| Teraspeed Labs
| http://www.teraspeedlabs.com
[IBIS Ver]  4.0
[File Name] ev12as350a.ibs
[File Rev]  3.0
[Source]  Created by Teraspeed Labs
[Date]   02/10/2017
[Notes]   Quality Check of this IBIS model: Model Passes IBIS Check
   Model parses into ICX IS. Simulation done with Hyperlynx.
   1. MIN TYP MAX information is based on Temperature and
   Voltage characteristics only.
   2. Package data gained using Tektronix IConnect Software.
[Disclaimer]
| Use: Teraspeed Labs  ("Teraspeed") has
| licensed IBIS models to specific integrated circuit
| suppliers ("IC Vendors") for use and distribution as
| follows: Each IC Vendor may use IBIS Models, and distribute
| them to IC Vendor's customers to use solely for developing
| printed circuit board designs. Users of this model may
| modify the IBIS model to suit its specific applications but
| rights to derivative works and such modifications shall belong
| to Teraspeed. No other distribution of these materials is
| permitted.
| DISCLAIMER OF WARRANTY: UNLESS OTHERWISE AGREED TO IN WRITING
| TERASPEED DISCLAIMS AND USER WAIVES ALL WARRANTIES, EXPRESS
| OR IMPLIED, INCLUDING WARRANTIES OF MERCHANTABILITY AND
| FITNESS FOR A PARTICULAR PURPOSE. IN NO EVENT SHALL
| TERASPEED BE LIABLE FOR ANY DIRECT OR INDIRECT DAMAGES,
| WHETHER IN CONTRACT OR TORT, INCLUDING, WITHOUT LIMITATION,
| LOST PROFITS, BUSINESS INTERRUPTION, OR LOST INFORMATION
| ARISING OUT OF THE USE OF OR THE INABILITY TO USE THE MODEL,
| EVEN IF TERASPEED HAS BEEN ADVISED OF THE POSSIBILITY OF SUCH
| DAMAGES.
[Copyright]
| This file is the legal property of Teraspeed Labs Copyright(c) 2017.
| All other rights are reserved.
[Component]   EV12AS350A
[Manufacturer] e2v semiconductors
| Data Sheet: 1160DX-December 15
[Package]
| EBGA380 RoHS
| variable   typ   min   max
R_pkg  1.099E-02  6.371E-03  1.748E-02
L_pkg  2.017E-09  7.430E-10  5.787E-09
C_pkg  7.766E-13  4.120E-13  1.913E-12
[Pin] signal_name   model_name   R_pin   L_pin   C_pin
A1   GND   GND   1.748E-02   7.430E-10   4.120E-13
A2   VCCD   POWER   1.660E-02   7.430E-10   4.120E-13
A3   ABP   lvds_out   1.577E-02   5.787E-09   1.913E-12
A4   ADR   lvds_out   1.499E-02   5.500E-09   1.818E-12
A5   AIR   lvds_out   1.426E-02   5.234E-09   1.730E-12
A6   GND   GND   1.360E-02   7.430E-10   4.120E-13
A7   CMIREFAB   POWER   1.301E-02   7.430E-10   4.120E-13
A8   CMIREFCD   POWER   1.251E-02   7.430E-10   4.120E-13
A9   GND   GND   1.209E-02   7.430E-10   4.120E-13
A10   GND   GND   1.177E-02   7.430E-10   4.120E-13
A11   GND   GND   1.155E-02   7.430E-10   4.120E-13
A12   VIN   analog   1.144E-02   7.430E-10   4.120E-13
A13   VINN   analog   1.144E-02   7.430E-10   4.120E-13
A14   GND   GND   1.155E-02   7.430E-10   4.120E-13
A15   GND   GND   1.177E-02   7.430E-10   4.120E-13
A16   GND   GND   1.209E-02   7.430E-10   4.120E-13
A17   NC   NC   1.251E-02   7.430E-10   4.120E-13
A18   NC   NC   1.301E-02   7.430E-10   4.120E-13
A19   GND   GND   1.360E-02   7.430E-10   4.120E-13
A20   DIR   lvds_out   1.426E-02   5.234E-09   1.730E-12
A21   DDR   lvds_out   1.499E-02   5.500E-09   1.818E-12
A22   DBP   lvds_out   1.577E-02   5.787E-09   1.913E-12
A23   VCCD   POWER   1.660E-02   7.430E-10   4.120E-13
A24   GND   GND   1.748E-02   7.430E-10   4.120E-13
B1   GND   GND   1.660E-02   7.430E-10   4.120E-13
B2   VCCD   POWER   1.568E-02   7.430E-10   4.120E-13
B3   ABPN   lvds_out   1.481E-02   5.435E-09   1.797E-12
B4   ADRN   lvds_out   1.398E-02   5.131E-09   1.696E-12
B5   AIRN   lvds_out   1.321E-02   4.849E-09   1.603E-12
B6   GND   GND   1.251E-02   7.430E-10   4.120E-13
B7   GND   GND   1.188E-02   7.430E-10   4.120E-13
B8   GND   GND   1.133E-02   7.430E-10   4.120E-13
B9   GND   GND   1.088E-02   7.430E-10   4.120E-13
B10   GND   GND   1.053E-02   7.430E-10   4.120E-13
B11   GND   GND   1.030E-02   7.430E-10   4.120E-13
B12   GND   GND   1.018E-02   7.430E-10   4.120E-13
B13   GND   GND   1.018E-02   7.430E-10   4.120E-13
B14   GND   GND   1.030E-02   7.430E-10   4.120E-13
B15   GND   GND   1.053E-02   7.430E-10   4.120E-13
B16   GND   GND   1.088E-02   7.430E-10   4.120E-13
B17   GND   GND   1.133E-02   7.430E-10   4.120E-13
B18   GND   GND   1.188E-02   7.430E-10   4.120E-13
B19   GND   GND   1.251E-02   7.430E-10   4.120E-13
B20   DIRN   lvds_out   1.321E-02   4.849E-09   1.603E-12
B21   DDRN   lvds_out   1.398E-02   5.131E-09   1.696E-12
B22   DBPN   lvds_out   1.481E-02   5.435E-09   1.797E-12
B23   VCCD   POWER   1.568E-02   7.430E-10   4.120E-13
B24   GND   GND   1.660E-02   7.430E-10   4.120E-13
C1   A11   lvds_out   1.577E-02   5.787E-09   1.913E-12
C2   A11N   lvds_out   1.481E-02   5.435E-09   1.797E-12
C3   VCCD   POWER   1.389E-02   7.430E-10   4.120E-13
C4   GND   GND   1.301E-02   7.430E-10   4.120E-13
C5   VCCD   POWER   1.220E-02   7.430E-10   4.120E-13
C6   VCCD   POWER   1.144E-02   7.430E-10   4.120E-13
C7   GND   GND   1.077E-02   7.430E-10   4.120E-13
C8   GND   GND   1.018E-02   7.430E-10   4.120E-13
C9   GND   GND   9.683E-03   7.430E-10   4.120E-13
C10   GND   GND   9.301E-03   7.430E-10   4.120E-13
C11   GND   GND   9.040E-03   7.430E-10   4.120E-13
C12   GND   GND   8.907E-03   7.430E-10   4.120E-13
C13   GND   GND   8.907E-03   7.430E-10   4.120E-13
C14   GND   GND   9.040E-03   7.430E-10   4.120E-13
C15   GND   GND   9.301E-03   7.430E-10   4.120E-13
C16   GND   GND   9.683E-03   7.430E-10   4.120E-13
C17   GND   GND   1.018E-02   7.430E-10   4.120E-13
C18   GND   GND   1.077E-02   7.430E-10   4.120E-13
C19   VCCD   POWER   1.144E-02   7.430E-10   4.120E-13
C20   VCCD   POWER   1.220E-02   7.430E-10   4.120E-13
C21   GND   GND   1.301E-02   7.430E-10   4.120E-13
C22   VCCD   POWER   1.389E-02   7.430E-10   4.120E-13
C23   D11N   lvds_out   1.481E-02   5.435E-09   1.797E-12
C24   D11   lvds_out   1.577E-02   5.787E-09   1.913E-12
D1   A10   lvds_out   1.499E-02   5.500E-09   1.818E-12
D2   A10N   lvds_out   1.398E-02   5.131E-09   1.696E-12
D3   VCCD   POWER   1.301E-02   7.430E-10   4.120E-13
D4   GND   GND   1.209E-02   7.430E-10   4.120E-13
D5   VCCO1   POWER   1.122E-02   7.430E-10   4.120E-13
D6   VCCD   POWER   1.042E-02   7.430E-10   4.120E-13
D7   VCCD   POWER   9.683E-03   7.430E-10   4.120E-13
D8   GND   GND   9.040E-03   7.430E-10   4.120E-13
D9   GND   GND   8.499E-03   7.430E-10   4.120E-13
D10   GND   GND   8.077E-03   7.430E-10   4.120E-13
D11   GND   GND   7.787E-03   7.430E-10   4.120E-13
D12   GND   GND   7.639E-03   7.430E-10   4.120E-13
D13   GND   GND   7.639E-03   7.430E-10   4.120E-13
D14   GND   GND   7.787E-03   7.430E-10   4.120E-13
D15   GND   GND   8.077E-03   7.430E-10   4.120E-13
D16   GND   GND   8.499E-03   7.430E-10   4.120E-13
D17   GND   GND   9.040E-03   7.430E-10   4.120E-13
D18   VCCD   POWER   9.683E-03   7.430E-10   4.120E-13
D19   VCCD   POWER   1.042E-02   7.430E-10   4.120E-13
D20   VCCO1   POWER   1.122E-02   7.430E-10   4.120E-13
D21   GND   GND   1.209E-02   7.430E-10   4.120E-13
D22   VCCD   POWER   1.301E-02   7.430E-10   4.120E-13
D23   D10N   lvds_out   1.398E-02   5.131E-09   1.696E-12
D24   D10   lvds_out   1.499E-02   5.500E-09   1.818E-12
E1   A9   lvds_out   1.426E-02   5.234E-09   1.730E-12
E2   A9N   lvds_out   1.321E-02   4.849E-09   1.603E-12
E3   VCCO1   POWER   1.220E-02   7.430E-10   4.120E-13
E4   GNDO   GND   1.122E-02   7.430E-10   4.120E-13
E5   GNDO   GND   1.030E-02   7.430E-10   4.120E-13
E6   VCCO1   POWER   9.429E-03   7.430E-10   4.120E-13
E7   VCCD   POWER   8.637E-03   7.430E-10   4.120E-13
E8   GND   GND   7.933E-03   7.430E-10   4.120E-13
E9   GND   GND   7.336E-03   7.430E-10   4.120E-13
E10   GND   GND   6.865E-03   7.430E-10   4.120E-13
E11   GND   GND   6.539E-03   7.430E-10   4.120E-13
E12   GND   GND   6.371E-03   7.430E-10   4.120E-13
E13   GND   GND   6.371E-03   7.430E-10   4.120E-13
E14   GND   GND   6.539E-03   7.430E-10   4.120E-13
E15   GND   GND   6.865E-03   7.430E-10   4.120E-13
E16   GND   GND   7.336E-03   7.430E-10   4.120E-13
E17   GND   GND   7.933E-03   7.430E-10   4.120E-13
E18   VCCD   POWER   8.637E-03   7.430E-10   4.120E-13
E19   VCCO1   POWER   9.429E-03   7.430E-10   4.120E-13
E20   GNDO   GND   1.030E-02   7.430E-10   4.120E-13
E21   GNDO   GND   1.122E-02   7.430E-10   4.120E-13
E22   VCCO1   POWER   1.220E-02   7.430E-10   4.120E-13
E23   D9N   lvds_out   1.321E-02   4.849E-09   1.603E-12
E24   D9   lvds_out   1.426E-02   5.234E-09   1.730E-12
F1   A8   lvds_out   1.360E-02   4.992E-09   1.650E-12
F2   A8N   lvds_out   1.251E-02   4.591E-09   1.518E-12
F3   VCCO1   POWER   1.144E-02   7.430E-10   4.120E-13
F4   GNDO   GND   1.042E-02   7.430E-10   4.120E-13
F5   GNDO   GND   9.429E-03   7.430E-10   4.120E-13
F20   GNDO   GND   9.429E-03   7.430E-10   4.120E-13
F21   GNDO   GND   1.042E-02   7.430E-10   4.120E-13
F22   VCCO1   POWER   1.144E-02   7.430E-10   4.120E-13
F23   D8N   lvds_out   1.251E-02   4.591E-09   1.518E-12
F24   D8   lvds_out   1.360E-02   4.992E-09   1.650E-12
G1   A6   lvds_out   1.301E-02   4.776E-09   1.579E-12
G2   A6N   lvds_out   1.188E-02   4.359E-09   1.441E-12
G3   A7   lvds_out   1.077E-02   3.951E-09   1.306E-12
G4   A7N   lvds_out   9.683E-03   3.554E-09   1.175E-12
G5   GNDO   GND   8.637E-03   7.430E-10   4.120E-13
G20   GNDO   GND   8.637E-03   7.430E-10   4.120E-13
G21   D7N   lvds_out   9.683E-03   3.554E-09   1.175E-12
G22   D7   lvds_out   1.077E-02   3.951E-09   1.306E-12
G23   D6N   lvds_out   1.188E-02   4.359E-09   1.441E-12
G24   D6   lvds_out   1.301E-02   4.776E-09   1.579E-12
H1   A4   lvds_out   1.251E-02   4.591E-09   1.518E-12
H2   A4N   lvds_out   1.133E-02   4.159E-09   1.375E-12
H3   A5   lvds_out   1.018E-02   3.734E-09   1.235E-12
H4   A5N   lvds_out   9.040E-03   3.318E-09   1.097E-12
H5   VCCO1   POWER   7.933E-03   7.430E-10   4.120E-13
H20   VCCO1   POWER   7.933E-03   7.430E-10   4.120E-13
H21   D5N   lvds_out   9.040E-03   3.318E-09   1.097E-12
H22   D5   lvds_out   1.018E-02   3.734E-09   1.235E-12
H23   D4N   lvds_out   1.133E-02   4.159E-09   1.375E-12
H24   D4   lvds_out   1.251E-02   4.591E-09   1.518E-12
J1   A2   lvds_out   1.209E-02   4.438E-09   1.467E-12
J2   A2N   lvds_out   1.088E-02   3.993E-09   1.320E-12
J3   A3   lvds_out   9.683E-03   3.554E-09   1.175E-12
J4   A3N   lvds_out   8.499E-03   3.119E-09   1.031E-12
J5   GND   GND   7.336E-03   7.430E-10   4.120E-13
J20   GND   GND   7.336E-03   7.430E-10   4.120E-13
J21   D3N   lvds_out   8.499E-03   3.119E-09   1.031E-12
J22   D3   lvds_out   9.683E-03   3.554E-09   1.175E-12
J23   D2N   lvds_out   1.088E-02   3.993E-09   1.320E-12
J24   D2   lvds_out   1.209E-02   4.438E-09   1.467E-12
K1   A0   lvds_out   1.177E-02   4.320E-09   1.428E-12
K2   A0N   lvds_out   1.053E-02   3.866E-09   1.278E-12
K3   A1   lvds_out   9.301E-03   3.413E-09   1.128E-12
K4   A1N   lvds_out   8.077E-03   2.964E-09   9.799E-13
K5   VCCD   POWER   6.865E-03   7.430E-10   4.120E-13
K20   VCCD   POWER   6.865E-03   7.430E-10   4.120E-13
K21   D1N   lvds_out   8.077E-03   2.964E-09   9.799E-13
K22   D1   lvds_out   9.301E-03   3.413E-09   1.128E-12
K23   D0N   lvds_out   1.053E-02   3.866E-09   1.278E-12
K24   D0   lvds_out   1.177E-02   4.320E-09   1.428E-12
L1   GND   GND   1.155E-02   7.430E-10   4.120E-13
L2   GND   GND   1.030E-02   7.430E-10   4.120E-13
L3   NC   NC   9.040E-03   7.430E-10   4.120E-13
L4   GND   GND   7.787E-03   7.430E-10   4.120E-13
L5   VCCD   POWER   6.539E-03   7.430E-10   4.120E-13
L20   VCCD   POWER   6.539E-03   7.430E-10   4.120E-13
L21   GND   GND   7.787E-03   7.430E-10   4.120E-13
L22   NC   NC   9.040E-03   7.430E-10   4.120E-13
L23   GND   GND   1.030E-02   7.430E-10   4.120E-13
L24   GND   GND   1.155E-02   7.430E-10   4.120E-13
M1   VCCA   POWER   1.144E-02   7.430E-10   4.120E-13
M2   GND   GND   1.018E-02   7.430E-10   4.120E-13
M3   VCCA   POWER   8.907E-03   7.430E-10   4.120E-13
M4   GND   GND   7.639E-03   7.430E-10   4.120E-13
M5   VCCD   POWER   6.371E-03   7.430E-10   4.120E-13
M20   VCCD   POWER   6.371E-03   7.430E-10   4.120E-13
M21   GND   GND   7.639E-03   7.430E-10   4.120E-13
M22   VCCA   POWER   8.907E-03   7.430E-10   4.120E-13
M23   GND   GND   1.018E-02   7.430E-10   4.120E-13
M24   VCCA   POWER   1.144E-02   7.430E-10   4.120E-13
N1   VCCA   POWER   1.144E-02   7.430E-10   4.120E-13
N2   GND   GND   1.018E-02   7.430E-10   4.120E-13
N3   VCCA   POWER   8.907E-03   7.430E-10   4.120E-13
N4   GND   GND   7.639E-03   7.430E-10   4.120E-13
N5   VCCD   POWER   6.371E-03   7.430E-10   4.120E-13
N20   VCCD   POWER   6.371E-03   7.430E-10   4.120E-13
N21   GND   GND   7.639E-03   7.430E-10   4.120E-13
N22   VCCA   POWER   8.907E-03   7.430E-10   4.120E-13
N23   GND   GND   1.018E-02   7.430E-10   4.120E-13
N24   VCCA   POWER   1.144E-02   7.430E-10   4.120E-13
P1   GND   GND   1.155E-02   7.430E-10   4.120E-13
P2   GND   GND   1.030E-02   7.430E-10   4.120E-13
P3   NC   NC   9.040E-03   7.430E-10   4.120E-13
P4   GND   GND   7.787E-03   7.430E-10   4.120E-13
P5   VCCD   POWER   6.539E-03   7.430E-10   4.120E-13
P20   VCCD   POWER   6.539E-03   7.430E-10   4.120E-13
P21   GND   GND   7.787E-03   7.430E-10   4.120E-13
P22   NC   NC   9.040E-03   7.430E-10   4.120E-13
P23   GND   GND   1.030E-02   7.430E-10   4.120E-13
P24   GND   GND   1.155E-02   7.430E-10   4.120E-13
R1   B0   lvds_out   1.177E-02   4.320E-09   1.428E-12
R2   B0N   lvds_out   1.053E-02   3.866E-09   1.278E-12
R3   B1   lvds_out   9.301E-03   3.413E-09   1.128E-12
R4   B1N   lvds_out   8.077E-03   2.964E-09   9.799E-13
R5   VCCD   POWER   6.865E-03   7.430E-10   4.120E-13
R20   VCCD   POWER   6.865E-03   7.430E-10   4.120E-13
R21   C1N   lvds_out   8.077E-03   2.964E-09   9.799E-13
R22   C1   lvds_out   9.301E-03   3.413E-09   1.128E-12
R23   C0N   lvds_out   1.053E-02   3.866E-09   1.278E-12
R24   C0   lvds_out   1.177E-02   4.320E-09   1.428E-12
T1   B2   lvds_out   1.209E-02   4.438E-09   1.467E-12
T2   B2N   lvds_out   1.088E-02   3.993E-09   1.320E-12
T3   B3   lvds_out   9.683E-03   3.554E-09   1.175E-12
T4   B3N   lvds_out   8.499E-03   3.119E-09   1.031E-12
T5   GND   GND   7.336E-03   7.430E-10   4.120E-13
T20   GND   GND   7.336E-03   7.430E-10   4.120E-13
T21   C3N   lvds_out   8.499E-03   3.119E-09   1.031E-12
T22   C3   lvds_out   9.683E-03   3.554E-09   1.175E-12
T23   C2N   lvds_out   1.088E-02   3.993E-09   1.320E-12
T24   C2   lvds_out   1.209E-02   4.438E-09   1.467E-12
U1   B4   lvds_out   1.251E-02   4.591E-09   1.518E-12
U2   B4N   lvds_out   1.133E-02   4.159E-09   1.375E-12
U3   B5   lvds_out   1.018E-02   3.734E-09   1.235E-12
U4   B5N   lvds_out   9.040E-03   3.318E-09   1.097E-12
U5   VCCO1   POWER   7.933E-03   7.430E-10   4.120E-13
U20   VCCO1   POWER   7.933E-03   7.430E-10   4.120E-13
U21   C5N   lvds_out   9.040E-03   3.318E-09   1.097E-12
U22   C5   lvds_out   1.018E-02   3.734E-09   1.235E-12
U23   C4N   lvds_out   1.133E-02   4.159E-09   1.375E-12
U24   C4   lvds_out   1.251E-02   4.591E-09   1.518E-12
V1   B6   lvds_out   1.301E-02   4.776E-09   1.579E-12
V2   B6N   lvds_out   1.188E-02   4.359E-09   1.441E-12
V3   B7   lvds_out   1.077E-02   3.951E-09   1.306E-12
V4   B7N   lvds_out   9.683E-03   3.554E-09   1.175E-12
V5   GNDO   GND   8.637E-03   7.430E-10   4.120E-13
V20   GNDO   GND   8.637E-03   7.430E-10   4.120E-13
V21   C7N   lvds_out   9.683E-03   3.554E-09   1.175E-12
V22   C7   lvds_out   1.077E-02   3.951E-09   1.306E-12
V23   C6N   lvds_out   1.188E-02   4.359E-09   1.441E-12
V24   C6   lvds_out   1.301E-02   4.776E-09   1.579E-12
W1   B8   lvds_out   1.360E-02   4.992E-09   1.650E-12
W2   B8N   lvds_out   1.251E-02   4.591E-09   1.518E-12
W3   VCCO1   POWER   1.144E-02   7.430E-10   4.120E-13
W4   GNDO   GND   1.042E-02   7.430E-10   4.120E-13
W5   GNDO   GND   9.429E-03   7.430E-10   4.120E-13
W20   GNDO   GND   9.429E-03   7.430E-10   4.120E-13
W21   GNDO   GND   1.042E-02   7.430E-10   4.120E-13
W22   VCCO1   POWER   1.144E-02   7.430E-10   4.120E-13
W23   C8N   lvds_out   1.251E-02   4.591E-09   1.518E-12
W24   C8   lvds_out   1.360E-02   4.992E-09   1.650E-12
Y1   B9   lvds_out   1.426E-02   5.234E-09   1.730E-12
Y2   B9N   lvds_out   1.321E-02   4.849E-09   1.603E-12
Y3   VCCO1   POWER   1.220E-02   7.430E-10   4.120E-13
Y4   GNDO   GND   1.122E-02   7.430E-10   4.120E-13
Y5   GNDO   GND   1.030E-02   7.430E-10   4.120E-13
Y6   VCCO1   POWER   9.429E-03   7.430E-10   4.120E-13
Y7   VCCD   POWER   8.637E-03   7.430E-10   4.120E-13
Y8   GND   GND   7.933E-03   7.430E-10   4.120E-13
Y9   GND   GND   7.336E-03   7.430E-10   4.120E-13
Y10   VCCD   POWER   6.865E-03   7.430E-10   4.120E-13
Y11   VCCD   POWER   6.539E-03   7.430E-10   4.120E-13
Y12   GND   GND   6.371E-03   7.430E-10   4.120E-13
Y13   GND   GND   6.371E-03   7.430E-10   4.120E-13
Y14   VCCD   POWER   6.539E-03   7.430E-10   4.120E-13
Y15   VCCD   POWER   6.865E-03   7.430E-10   4.120E-13
Y16   GND   GND   7.336E-03   7.430E-10   4.120E-13
Y17   GND   GND   7.933E-03   7.430E-10   4.120E-13
Y18   VCCD   POWER   8.637E-03   7.430E-10   4.120E-13
Y19   VCCO1   POWER   9.429E-03   7.430E-10   4.120E-13
Y20   GNDO   GND   1.030E-02   7.430E-10   4.120E-13
Y21   GNDO   GND   1.122E-02   7.430E-10   4.120E-13
Y22   VCCO1   POWER   1.220E-02   7.430E-10   4.120E-13
Y23   C9N   lvds_out   1.321E-02   4.849E-09   1.603E-12
Y24   C9   lvds_out   1.426E-02   5.234E-09   1.730E-12
AA1   B10   lvds_out   1.499E-02   5.500E-09   1.818E-12
AA2   B10N   lvds_out   1.398E-02   5.131E-09   1.696E-12
AA3   VCCD   POWER   1.301E-02   7.430E-10   4.120E-13
AA4   GND   GND   1.209E-02   7.430E-10   4.120E-13
AA5   VCCO1   POWER   1.122E-02   7.430E-10   4.120E-13
AA6   VCCD   POWER   1.042E-02   7.430E-10   4.120E-13
AA7   VCCD   POWER   9.683E-03   7.430E-10   4.120E-13
AA8   GND   GND   9.040E-03   7.430E-10   4.120E-13
AA9   GND   GND   8.499E-03   7.430E-10   4.120E-13
AA10   VCCD   POWER   8.077E-03   7.430E-10   4.120E-13
AA11   VCCD   POWER   7.787E-03   7.430E-10   4.120E-13
AA12   GND   GND   7.639E-03   7.430E-10   4.120E-13
AA13   GND   GND   7.639E-03   7.430E-10   4.120E-13
AA14   VCCD   POWER   7.787E-03   7.430E-10   4.120E-13
AA15   VCCD   POWER   8.077E-03   7.430E-10   4.120E-13
AA16   GND   GND   8.499E-03   7.430E-10   4.120E-13
AA17   GND   GND   9.040E-03   7.430E-10   4.120E-13
AA18   VCCD   POWER   9.683E-03   7.430E-10   4.120E-13
AA19   VCCD   POWER   1.042E-02   7.430E-10   4.120E-13
AA20   VCCO1   POWER   1.122E-02   7.430E-10   4.120E-13
AA21   GND   GND   1.209E-02   7.430E-10   4.120E-13
AA22   VCCD   POWER   1.301E-02   7.430E-10   4.120E-13
AA23   C10N   lvds_out   1.398E-02   5.131E-09   1.696E-12
AA24   C10   lvds_out   1.499E-02   5.500E-09   1.818E-12
AB1   B11   lvds_out   1.577E-02   5.787E-09   1.913E-12
AB2   B11N   lvds_out   1.481E-02   5.435E-09   1.797E-12
AB3   VCCD   POWER   1.389E-02   7.430E-10   4.120E-13
AB4   GND   GND   1.301E-02   7.430E-10   4.120E-13
AB5   VCCD   POWER   1.220E-02   7.430E-10   4.120E-13
AB6   GND   GND   1.144E-02   7.430E-10   4.120E-13
AB7   VCCD   POWER   1.077E-02   7.430E-10   4.120E-13
AB8   GND   GND   1.018E-02   7.430E-10   4.120E-13
AB9   GND   GND   9.683E-03   7.430E-10   4.120E-13
AB10   VCCD   POWER   9.301E-03   7.430E-10   4.120E-13
AB11   VCCD   POWER   9.040E-03   7.430E-10   4.120E-13
AB12   GND   GND   8.907E-03   7.430E-10   4.120E-13
AB13   GND   GND   8.907E-03   7.430E-10   4.120E-13
AB14   VCCD   POWER   9.040E-03   7.430E-10   4.120E-13
AB15   VCCD   POWER   9.301E-03   7.430E-10   4.120E-13
AB16   GND   GND   9.683E-03   7.430E-10   4.120E-13
AB17   GND   GND   1.018E-02   7.430E-10   4.120E-13
AB18   VCCD   POWER   1.077E-02   7.430E-10   4.120E-13
AB19   GND   GND   1.144E-02   7.430E-10   4.120E-13
AB20   VCCD   POWER   1.220E-02   7.430E-10   4.120E-13
AB21   GND   GND   1.301E-02   7.430E-10   4.120E-13
AB22   VCCD   POWER   1.389E-02   7.430E-10   4.120E-13
AB23   C11N   lvds_out   1.481E-02   5.435E-09   1.797E-12
AB24   C11   lvds_out   1.577E-02   5.787E-09   1.913E-12
AC1   GND   GND   1.660E-02   7.430E-10   4.120E-13
AC2   VCCD   POWER   1.568E-02   7.430E-10   4.120E-13
AC3   BBPN   lvds_out   1.481E-02   5.435E-09   1.797E-12
AC4   BDRN   lvds_out   1.398E-02   5.131E-09   1.696E-12
AC5   BIRN   lvds_out   1.321E-02   4.849E-09   1.603E-12
AC6   GND   GND   1.251E-02   7.430E-10   4.120E-13
AC7   diodeC   GND   1.188E-02   7.430E-10   4.120E-13
AC8   NC   NC   1.133E-02   7.430E-10   4.120E-13
AC9   GND   GND   1.088E-02   7.430E-10   4.120E-13
AC10   SYNCN   sync_in   1.053E-02   3.866E-09   1.278E-12
AC11   GND   GND   1.030E-02   7.430E-10   4.120E-13
AC12   GND   GND   1.018E-02   7.430E-10   4.120E-13
AC13   GND   GND   1.018E-02   7.430E-10   4.120E-13
AC14   GND   GND   1.030E-02   7.430E-10   4.120E-13
AC15   *RST   in_pu   1.053E-02   3.866E-09   1.278E-12
AC16   *CS   in_pu   1.088E-02   3.993E-09   1.320E-12
AC17   MISO   spi_out   1.133E-02   4.159E-09   1.375E-12
AC18   VCCO2   POWER   1.188E-02   7.430E-10   4.120E-13
AC19   GND   GND   1.251E-02   7.430E-10   4.120E-13
AC20   CIRN   lvds_out   1.321E-02   4.849E-09   1.603E-12
AC21   CDRN   lvds_out   1.398E-02   5.131E-09   1.696E-12
AC22   CBPN   lvds_out   1.481E-02   5.435E-09   1.797E-12
AC23   VCCD   POWER   1.568E-02   7.430E-10   4.120E-13
AC24   GND   GND   1.660E-02   7.430E-10   4.120E-13
AD1   GND   GND   1.748E-02   7.430E-10   4.120E-13
AD2   VCCD   POWER   1.660E-02   7.430E-10   4.120E-13
AD3   BBP   lvds_out   1.577E-02   5.787E-09   1.913E-12
AD4   BDR   lvds_out   1.499E-02   5.500E-09   1.818E-12
AD5   BIR   lvds_out   1.426E-02   5.234E-09   1.730E-12
AD6   GND   GND   1.360E-02   7.430E-10   4.120E-13
AD7   diodeA   NC   1.301E-02   7.430E-10   4.120E-13
AD8   GND   GND   1.251E-02   7.430E-10   4.120E-13
AD9   GND   GND   1.209E-02   7.430E-10   4.120E-13
AD10   SYNCP   sync_in   1.177E-02   4.320E-09   1.428E-12
AD11   GND   GND   1.155E-02   7.430E-10   4.120E-13
AD12   CLK   clk_in   1.144E-02   4.200E-09   1.388E-12
AD13   CLKN   clk_in   1.144E-02   4.200E-09   1.388E-12
AD14   GND   GND   1.155E-02   7.430E-10   4.120E-13
AD15   NC   NC   1.177E-02   7.430E-10   4.120E-13
AD16   SCLK   spi_in   1.209E-02   4.438E-09   1.467E-12
AD17   MOSI   spi_in   1.251E-02   4.591E-09   1.518E-12
AD18   VCCO2   POWER   1.301E-02   7.430E-10   4.120E-13
AD19   GND   GND   1.360E-02   7.430E-10   4.120E-13
AD20   CIR   lvds_out   1.426E-02   5.234E-09   1.730E-12
AD21   CDR   lvds_out   1.499E-02   5.500E-09   1.818E-12
AD22   CBP   lvds_out   1.577E-02   5.787E-09   1.913E-12
AD23   VCCD   POWER   1.660E-02   7.430E-10   4.120E-13
AD24   GND   GND   1.748E-02   7.430E-10   4.120E-13
[Diff Pin] inv_pin vdiff tdelay_typ tdelay_min tdelay_max
AD12   AD13   158mV   NA   NA   NA
AD10   AC10   100mV   NA   NA   NA
K1   K2   NA   NA   NA   NA
K3   K4   NA   NA   NA   NA
J1   J2   NA   NA   NA   NA
J3   J4   NA   NA   NA   NA
H1   H2   NA   NA   NA   NA
H3   H4   NA   NA   NA   NA
G1   G2   NA   NA   NA   NA
G3   G4   NA   NA   NA   NA
F1   F2   NA   NA   NA   NA
E1   E2   NA   NA   NA   NA
D1   D2   NA   NA   NA   NA
C1   C2   NA   NA   NA   NA
A3   B3   NA   NA   NA   NA
A5   B5   NA   NA   NA   NA
A4   B4   NA   NA   NA   NA
R1   R2   NA   NA   NA   NA
R3   R4   NA   NA   NA   NA
T1   T2   NA   NA   NA   NA
T3   T4   NA   NA   NA   NA
U1   U2   NA   NA   NA   NA
U3   U4   NA   NA   NA   NA
V1   V2   NA   NA   NA   NA
V3   V4   NA   NA   NA   NA
W1   W2   NA   NA   NA   NA
Y1   Y2   NA   NA   NA   NA
AA1   AA2   NA   NA   NA   NA
AB1   AB2   NA   NA   NA   NA
AD3   AC3   NA   NA   NA   NA
AD5   AC5   NA   NA   NA   NA
AD4   AC4   NA   NA   NA   NA
R24   R23   NA   NA   NA   NA
R22   R21   NA   NA   NA   NA
T24   T23   NA   NA   NA   NA
T22   T21   NA   NA   NA   NA
U24   U23   NA   NA   NA   NA
U22   U21   NA   NA   NA   NA
V24   V23   NA   NA   NA   NA
V22   V21   NA   NA   NA   NA
W24   W23   NA   NA   NA   NA
Y24   Y23   NA   NA   NA   NA
AA24   AA23   NA   NA   NA   NA
AB24   AB23   NA   NA   NA   NA
AD22   AC22   NA   NA   NA   NA
AD20   AC20   NA   NA   NA   NA
AD21   AC21   NA   NA   NA   NA
K24   K23   NA   NA   NA   NA
K22   K21   NA   NA   NA   NA
J24   J23   NA   NA   NA   NA
J22   J21   NA   NA   NA   NA
H24   H23   NA   NA   NA   NA
H22   H21   NA   NA   NA   NA
G24   G23   NA   NA   NA   NA
G22   G21   NA   NA   NA   NA
F24   F23   NA   NA   NA   NA
E24   E23   NA   NA   NA   NA
D24   D23   NA   NA   NA   NA
C24   C23   NA   NA   NA   NA
A22   B22   NA   NA   NA   NA
A20   B20   NA   NA   NA   NA
A21   B21   NA   NA   NA   NA
[Series Pin Mapping] pin_2 model_name function_table_group
AD12   AD13   100ohm
AD10   AC10   100ohm
[Model selector] lvds_out
lvds_lo_swing   lvds out,reduced swing |default
lvds_norm_swing   lvds out,normal swing
[Model] 100ohm
Model_type  Series
C_comp   0  0  0
[Voltage Range]  1.80   1.70   1.90
[Temperature Range]  25   110   -40
[R series]   100   90   110
[Model] analog
Model_type Terminator
C_comp   0  0  0
| variable   typ   min   max
[Voltage Range]   4.80V   4.70V   4.90V
[POWER Clamp Reference]  4.80V   4.70V   4.90V
[GND Clamp Reference]   0.00V   0.00V   0.00V
[Temperature Range]  25   110   -40
| Models and submodels in the file (9): clk_in (Input), in_pu (Input), spi_in (Input), sync_in (Input), lvds_lo_swing (Output), lvds_norm_swing (Output), spi_out (Output), 100ohm (Series), analog (Terminator)
